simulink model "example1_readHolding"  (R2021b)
settings: Solver=FixedStepDiscrete  StartTime=0.0  StopTime=10.0  FixedStep=0.5  RelTol=1e-3
libraries: ModbusServerLib x3

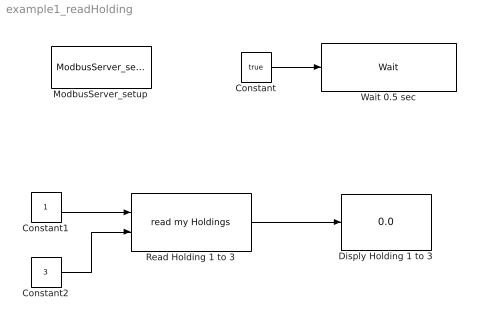
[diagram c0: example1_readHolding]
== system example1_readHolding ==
  Constant : Constant  Value=true
  Constant1 : Constant
  Constant2 : Constant  Value=3
  Disply Holding 1 to 3 : Display
  ModbusServer_setup : ModbusServerLib/ModbusServer_setup  g1_cmbPortName="\"COM5\""  g2_cmbModbusType="\"Modbus RTU\""  g3_chkIgnoreServerID=off  g4_ObjectID=0  g5_ServerID=[1 2 3 4 5 ]  g30_TCPPort=502  g6_chkSupportDINCoil1to4=on  g7_HoldingRegsSeg1to4=[ 1,30 ; 35, 56]  g8_InputRegsSeg1to4=[1 44; 78 89]  g9_CoilSeg1to4=[1 44; 78 89]  g10_DiscreteSeg1to4=[1 44; 78 89]  g11_chkUseHoldingRegstoReplace1to4=off  g12_chkEnableWD1to4=off  g13_chkUseReadonlyRegs4WD1to4=off  g14_WDAddr1to4=1  g15_cmbWDType1to4=0  g16_WDPeriod1to4=20  g17_WDPreset1to4=20  g18_chkSupportDINCoil5=on  g19_HoldingRegsSeg5=[ 1,30 ; 35, 56]  g20_InputRegsSeg5=[1 44; 78 89]  g21_CoilSeg5=[1 44; 78 89]  g22_DiscreteSeg5=[1 44; 78 89]  g23_chkUseHoldingRegstoReplace5=off  g24_chkEnableWD5=off  g25_chkUseReadonlyRegs4WD5=off  g26_WDAddr5=1  g27_cmbWDType5=0  g28_WDPeriod5=20  g29_WDPreset5=20
  Read Holding 1 to 3 : ModbusServerLib/read my Holdings  g_ObjID=0  g_endian=big-endian  g_OutputDataType=uint16  g_DeviceNum=1
  Wait 0.5 sec : ModbusServerLib/Wait  Waitms=500
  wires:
  Constant/1 -> Wait 0.5 sec/1
  Read Holding 1 to 3/1 -> Disply Holding 1 to 3/1
  Constant1/1 -> Read Holding 1 to 3/1
  Constant2/1 -> Read Holding 1 to 3/2
